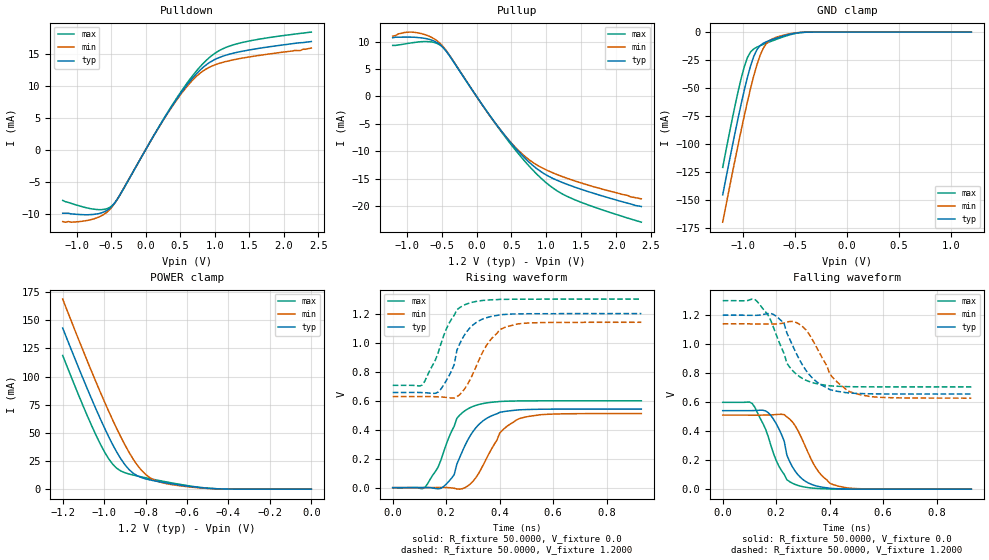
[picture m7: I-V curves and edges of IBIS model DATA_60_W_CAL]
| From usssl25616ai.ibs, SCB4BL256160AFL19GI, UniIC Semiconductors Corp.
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|   Model DATA_60_W_CAL
[Model]  DATA_60_W_CAL
Model_type I/O
Polarity   Non-Inverting
Enable   Active-High
Vinl =   0.3800V
Vinh =   0.8200V
Vmeas =  0.6000V
Cref =   5.0000pF
Rref =   50.0000
Vref =   0.6000V
C_comp   1.7430pF   1.7110pF   1.7640pF
[Temperature Range]   25.0000   85.0000   -40.0000
[Voltage Range]   1.2000V   1.1400V   1.3000V
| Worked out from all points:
|   slope of the pulldown table from 0 to 0.18 V, typ, clamps not added: 54.2 ohm
|   slope of the pullup table from 0 to 0.18 V, typ, clamps not added: 54.6 ohm
|   GND clamp passes 1 mA (typ) near -0.50 V on its own axis
|   POWER clamp passes 1 mA (typ) near -0.51 V on its own axis
|   rising waveform, R_fixture 50.0000, V_fixture 0.0: 20-80 % time 88.7ps typ, 95.6ps min, 78ps max; typ from 0 V to 0.542 V
|   rising waveform, R_fixture 50.0000, V_fixture 1.2000: 20-80 % time 75.5ps typ, 89.8ps min, 83.9ps max; typ from 0.656 V to 1.2 V
|   falling waveform, R_fixture 50.0000, V_fixture 0.0: 20-80 % time 72.3ps typ, 86.9ps min, 80.2ps max; typ from 0.542 V to 0 V
|   falling waveform, R_fixture 50.0000, V_fixture 1.2000: 20-80 % time 98.8ps typ, 99.9ps min, 83.4ps max; typ from 1.2 V to 0.656 V
[Pulldown]
|Voltage   I(typ)   I(min)   I(max)
-1.2V     -9.9mA     -11.2mA    -7.9mA
-760mV    -10.09mA   -10.82mA   -9.253mA
-600mV    -9.689mA   -10.06mA   -9.296mA
-480mV    -8.742mA   -8.84mA    -8.678mA
-360mV    -6.833mA   -6.817mA   -6.86mA
80mV      1.497mA    1.485mA    1.516mA
360mV     6.436mA    6.35mA     6.554mA
600mV     10.13mA    9.89mA     10.41mA
840mV     12.94mA    12.36mA    13.55mA
1.04V     14.29mA    13.4mA     15.32mA
1.28V     15.11mA    14.07mA    16.42mA
2.4V      16.9mA     15.9mA     18.38mA
[Pullup]
|Voltage   I(typ)   I(min)   I(max)
-1.2V     10.7mA     11mA       9.3mA
-1V       10.81mA    11.7mA     9.62mA
-800mV    10.69mA    11.49mA    9.97mA
-600mV    10.05mA    10.46mA    9.813mA
-480mV    8.939mA    9.104mA    8.947mA
120mV     -2.222mA   -2.253mA   -2.247mA
360mV     -6.382mA   -6.392mA   -6.531mA
600mV     -10.04mA   -9.855mA   -10.46mA
840mV     -12.96mA   -12.33mA   -13.89mA
1.08V     -14.89mA   -13.88mA   -16.59mA
1.32V     -16.16mA   -15.05mA   -18.38mA
2.36V     -20.1mA    -18.7mA    -22.96mA
[GND_clamp]
|Voltage   I(typ)   I(min)   I(max)
-1.2V     -145.3mA   -169.7mA   -120.8mA
-1.11V    -103.1mA   -127.3mA   -78.51mA
-1.05V    -76.2mA    -100.1mA   -52.43mA
-990mV    -51.2mA    -74mA      -30.39mA
-960mV    -39.9mA    -61.63mA   -22.48mA
-900mV    -21.67mA   -39mA      -15mA
-870mV    -15.78mA   -29.25mA   -13.45mA
-810mV    -10.04mA   -14.72mA   -11.07mA
-750mV    -7.557mA   -7.71mA    -8.865mA
-600mV    -3.111mA   -2.463mA   -3.804mA
-420mV    -215.4uA   -156.1uA   -235uA
1.2V      1.597nA    5.589nA    1.463nA
[POWER_clamp]
|Voltage   I(typ)   I(min)   I(max)
-1.2V     143mA      168.8mA    118.7mA
-1.06V    79.88mA    104.3mA    56.26mA
-1.02V    63.08mA    86.79mA    40.63mA
-980mV    47.32mA    69.97mA    27.48mA
-940mV    33.2mA     54.05mA    18.67mA
-880mV    17.43mA    32.78mA    13.45mA
-840mV    11.87mA    21.34mA    11.69mA
-800mV    9.133mA    13.1mA     10.12mA
-720mV    6.135mA    5.731mA    7.166mA
-560mV    1.838mA    1.456mA    2.161mA
-420mV    156.9uA    132.7uA    153uA
0V        1.597nA    1.927nA    2.16nA
[Ramp]
| variable   typ   min   max
dV/dt_r  0.3250/88.8406p   0.3065/98.1936p   0.3593/81.8602p
dV/dt_f  0.3264/93.6061p   0.3073/0.1022n   0.3569/86.8204p
R_load = 50.0000
[Rising Waveform]
R_fixture= 50.0000
V_fixture= 0.0
V_fixture_min= 0.0
V_fixture_max= 0.0
|time   V(typ)   V(min)   V(max)
0s        0V         0V         0V
120ps     1.169mV    198.4uV    701uV
170ps     -8.318mV   1.076mV    142.3mV
190ps     6.689mV    1.494mV    243.2mV
230ps     89.65mV    -4.192mV   423.2mV
240ps     162.2mV    -9.511mV   477.9mV
310ps     410.5mV    65.77mV    566.5mV
400ps     518.7mV    375.2mV    594mV
470ps     536mV      473.3mV    597.8mV
930ps     541.6mV    510.8mV    598.9mV
[Rising Waveform]
R_fixture= 50.0000
V_fixture= 1.2000
V_fixture_min= 1.1400
V_fixture_max= 1.3000
|time   V(typ)   V(min)   V(max)
0s        656mV      627.8mV    705.2mV
110ps     655.3mV    628.2mV    706.6mV
170ps     658.9mV    626mV      929.9mV
220ps     805mV      617.8mV    1.162V
230ps     848.4mV    617.3mV    1.188V
240ps     946.5mV    627.2mV    1.226V
280ps     1.082V     712.5mV    1.268V
350ps     1.171V     978.3mV    1.292V
420ps     1.194V     1.105V     1.298V
930ps     1.2V       1.14V      1.3V
[Falling Waveform]
R_fixture= 50.0000
V_fixture= 0.0
V_fixture_min= 0.0
V_fixture_max= 0.0
|time   V(typ)   V(min)   V(max)
0s        541.6mV    510.8mV    598.9mV
110ps     541.7mV    510.4mV    591.3mV
170ps     528mV      511.5mV    364mV
220ps     376.8mV    516.2mV    127.6mV
230ps     331.8mV    514mV      102.1mV
240ps     234.8mV    498.4mV    65.2mV
280ps     102.4mV    408.9mV    26.5mV
350ps     22.47mV    143mV      5.461mV
420ps     3.913mV    27.35mV    895.8uV
930ps     0V         0V         0V
[Falling Waveform]
R_fixture= 50.0000
V_fixture= 1.2000
V_fixture_min= 1.1400
V_fixture_max= 1.3000
|time   V(typ)   V(min)   V(max)
0s        1.2V       1.14V      1.3V
120ps     1.199V     1.139V     1.309V
170ps     1.211V     1.139V     1.2V
200ps     1.193V     1.139V     1.066V
230ps     1.14V      1.146V     934mV
250ps     1.037V     1.156V     842.9mV
330ps     777mV      1.049V     738.1mV
400ps     687mV      796.4mV    712.8mV
480ps     662.5mV    669.1mV    706.7mV
930ps     656mV      627.8mV    705.2mV
